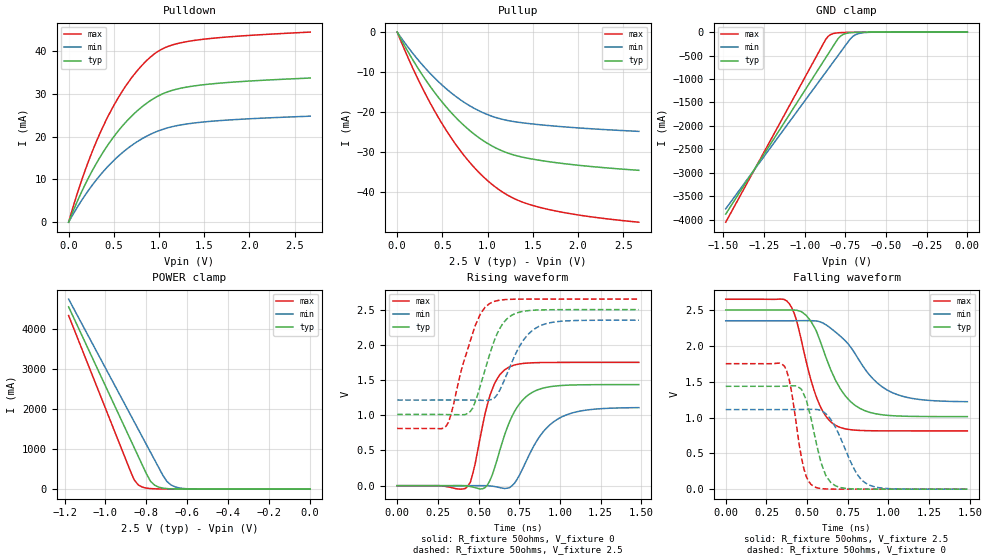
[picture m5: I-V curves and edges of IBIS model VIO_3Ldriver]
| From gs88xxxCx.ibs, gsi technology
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|  signals   DQA1-DQA9, DQB1-DQB9, DQC1-DQC9, DQD1-DQD9
[Model]   VIO_3Ldriver
Model_type   I/O
Polarity   Non-Inverting
Vinl  =   0.8v
Vinh  =   2.0v
Vmeas =   1.5v
Cref  =   0.0pF
Rref  =   50
Vref  =   1.5v
|  variable   typ   min   max
C_comp   3.0pF   2.5pF   3.5pF
|  variable   typ   min   max
[Temperature Range]   50   0   100
|  variable   typ   min   max
[Voltage Range]   2.5   2.35   2.65
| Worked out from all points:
|   slope of the pulldown table from 0 to 0.375 V, typ, clamps not added: 23.2 ohm
|   slope of the pullup table from 0 to 0.375 V, typ, clamps not added: 27 ohm
|   GND clamp passes 1 mA (typ) near -0.61 V on its own axis
|   POWER clamp passes 1 mA (typ) near -0.59 V on its own axis
|   rising waveform, R_fixture 50ohms, V_fixture 0: 20-80 % time 144ps typ, 184ps min, 107ps max; typ from 0 V to 1.44 V
|   rising waveform, R_fixture 50ohms, V_fixture 2.5: 20-80 % time 127ps typ, 147ps min, 132ps max; typ from 1.01 V to 2.5 V
|   falling waveform, R_fixture 50ohms, V_fixture 2.5: 20-80 % time 175ps typ, 241ps min, 133ps max; typ from 2.5 V to 1.01 V
|   falling waveform, R_fixture 50ohms, V_fixture 0: 20-80 % time 93ps typ, 136ps min, 72.9ps max; typ from 1.44 V to 0 V
[Pulldown]
| voltage   typ   min   max
0V        -354.4pA   -1.034nA   -211.5pA
108mV     5.444mA    3.903mA    7.511mA
216mV     10.22mA    7.345mA    14.05mA
324mV     14.39mA    10.36mA    19.71mA
432mV     18mA       12.99mA    24.6mA
540mV     21.12mA    15.26mA    28.8mA
675mV     24.37mA    17.62mA    33.18mA
810mV     26.98mA    19.51mA    36.68mA
945mV     28.99mA    20.96mA    39.34mA
1.134V    30.79mA    22.3mA     41.4mA
1.404V    31.95mA    23.26mA    42.59mA
2.673V    33.75mA    24.82mA    44.5mA
[Pullup]
| voltage (VDDQ-Vout)   typ   min   max
0V        284.9pA    1.042nA    119pA
243mV     -9.504mA   -7.26mA    -12.37mA
378mV     -14mA      -10.65mA   -18.28mA
513mV     -17.95mA   -13.59mA   -23.53mA
648mV     -21.37mA   -16.1mA    -28.13mA
783mV     -24.27mA   -18.18mA   -32.1mA
918mV     -26.66mA   -19.85mA   -35.45mA
1.053V    -28.56mA   -21.1mA    -38.2mA
1.296V    -30.81mA   -22.43mA   -41.71mA
1.566V    -32.07mA   -23.17mA   -43.83mA
2.025V    -33.39mA   -24.03mA   -45.87mA
2.673V    -34.61mA   -24.86mA   -47.6mA
[GND Clamp]
| voltage   typ   min   max
-1.485V   -3.884A    -3.771A    -4.056A
-885mV    -626.9mA   -926.9mA   -247.2mA
-870mV    -545.6mA   -856mA     -153.5mA
-855mV    -464.4mA   -785mA     -89.11mA
-825mV    -301.9mA   -643.2mA   -32.88mA
-795mV    -141.5mA   -501.4mA   -15.38mA
-780mV    -86.61mA   -430.5mA   -11.65mA
-750mV    -32.85mA   -288.8mA   -7.734mA
-705mV    -8.727mA   -95.28mA   -4.834mA
-660mV    -2.907mA   -24.97mA   -2.925mA
-555mV    -316.7uA   -1.176mA   -484.9uA
0V        -354.4pA   -1.034nA   -211.5pA
[POWER Clamp]
| voltage (VDDQ-Vout)   typ   min   max
-1.18V    4.545A     4.74A      4.328A
-880mV    1.258A     1.875A     474.1mA
-860mV    1.039A     1.684A     234.3mA
-840mV    820.4mA    1.493A     107.4mA
-820mV    601.5mA    1.302A     50.64mA
-780mV    197.3mA    920.5mA    14.28mA
-760mV    99.71mA    729.7mA    9.034mA
-720mV    26.23mA    348.2mA    4.898mA
-700mV    13.96mA    192.6mA    3.916mA
-660mV    4.495mA    57.55mA    2.579mA
-560mV    510.5uA    2.941mA    648.3uA
0V        285pA      1.042nA    119.1pA
[Ramp]
| voltage   typ   min   max
dV/dt_r   1.27/107p   1.05/135p   1.55/90p
dV/dt_f   1.26/107p   1.03/134p   1.51/89p
R_load  =   50ohms
[Rising Waveform]
C_fixture =   0.0pF
R_fixture =   50ohms
V_fixture =   0
| Time   V(typ)   V(min)   V(max)
0s        4.806nV    17.7nV     2.239nV
435ps     -6.875mV   506.6uV    -4.305mV
480ps     -28.91mV   711.5uV    318mV
555ps     9.634mV    -684.6uV   1.155V
615ps     374.9mV    -19.37mV   1.518V
690ps     903.2mV    -29.14mV   1.688V
810ps     1.295V     431.7mV    1.742V
900ps     1.387V     772.4mV    1.749V
990ps     1.419V     950.1mV    1.75V
1.485ns   1.435V     1.108V     1.751V
[Rising Waveform]
C_fixture =   0.0pF
R_fixture =   50ohms
V_fixture =   2.5
V_fixture_min =  2.35
V_fixture_max =  2.65
| Time   V(typ)   V(min)   V(max)
0s        1.012V     1.216V     812.7mV
300ps     1.01V      1.216V     843.9mV
450ps     1.056V     1.216V     2.061V
510ps     1.412V     1.213V     2.432V
570ps     1.877V     1.219V     2.59V
615ps     2.162V     1.293V     2.627V
675ps     2.369V     1.588V     2.644V
765ps     2.472V     2.028V     2.649V
870ps     2.495V     2.261V     2.65V
1.485ns   2.5V       2.35V      2.65V
[Falling Waveform]
C_fixture =   0.0pF
R_fixture =   50ohms
V_fixture =   2.5
V_fixture_min =  2.35
V_fixture_max =  2.65
| Time   V(typ)   V(min)   V(max)
0s        2.5V       2.35V      2.65V
390ps     2.5V       2.35V      2.591V
435ps     2.498V     2.35V      2.356V
555ps     2.217V     2.347V     1.299V
615ps     1.845V     2.295V     1.02V
675ps     1.519V     2.191V     890.9mV
795ps     1.169V     1.89V      823.7mV
900ps     1.063V     1.552V     815.1mV
1.005ns   1.028V     1.368V     813.5mV
1.485ns   1.012V     1.221V     813mV
[Falling Waveform]
C_fixture =   0.0pF
R_fixture =   50ohms
V_fixture =   0
| Time   V(typ)   V(min)   V(max)
0s        1.435V     1.111V     1.751V
360ps     1.437V     1.11V      1.719V
405ps     1.443V     1.111V     1.356V
465ps     1.395V     1.112V     443.4mV
540ps     820mV      1.113V     39.52mV
615ps     190.7mV    1.052V     3.231mV
675ps     46.11mV    860.4mV    543.4uV
795ps     2.9mV      257.8mV    38.32uV
870ps     596.6uV    70.66mV    9.691uV
1.485ns   1.862uV    9.427uV    728.4nV
